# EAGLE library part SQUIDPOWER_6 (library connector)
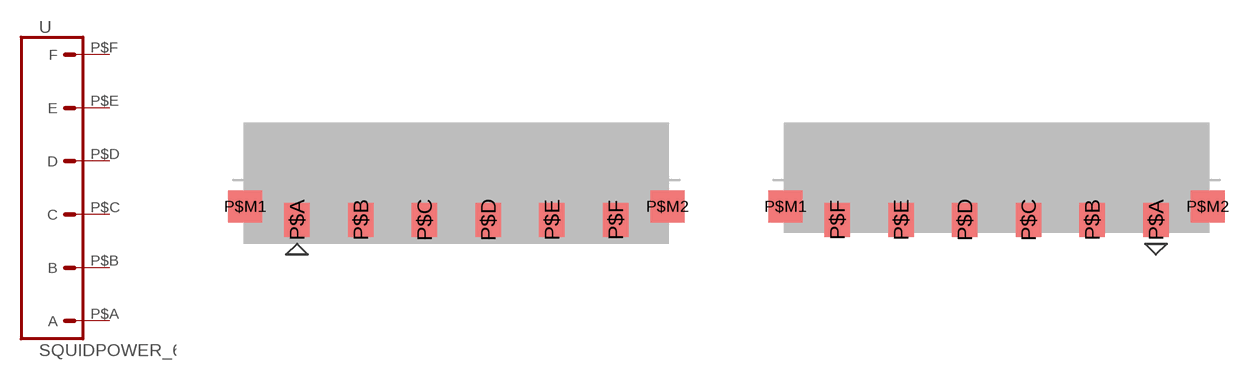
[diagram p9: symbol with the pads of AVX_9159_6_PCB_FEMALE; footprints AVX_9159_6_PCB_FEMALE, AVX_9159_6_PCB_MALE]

Designator prefix -

## SQUIDPOWER_6FEMALE  [AVX_9159_6_PCB_FEMALE]
P$A  A  pas
P$B  B  pas
P$C  C  pas
P$D  D  pas
P$E  E  pas
P$F  F  pas

## SQUIDPOWER_6MALE  [AVX_9159_6_PCB_MALE]
Pads as for AVX_9159_6_PCB_FEMALE

## Footprint AVX_9159_6_PCB_FEMALE (pad centres in mm)
smd 1.2 x 1.6: P$A -7.5,-1.88; P$B -4.5,-1.88; P$C -1.5,-1.88; P$D 1.5,-1.88; P$E 4.5,-1.88; P$F 7.5,-1.88
smd 1.6 x 1.5: P$M1 -9.935,-1.25; P$M2 9.935,-1.25

## Footprint AVX_9159_6_PCB_MALE (pad centres in mm)
smd 1.2 x 1.6: P$A 7.5,-1.88; P$B 4.5,-1.88; P$C 1.5,-1.88; P$D -1.5,-1.88; P$E -4.5,-1.88; P$F -7.5,-1.88
smd 1.6 x 1.5: P$M1 -9.935,-1.25; P$M2 9.935,-1.25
